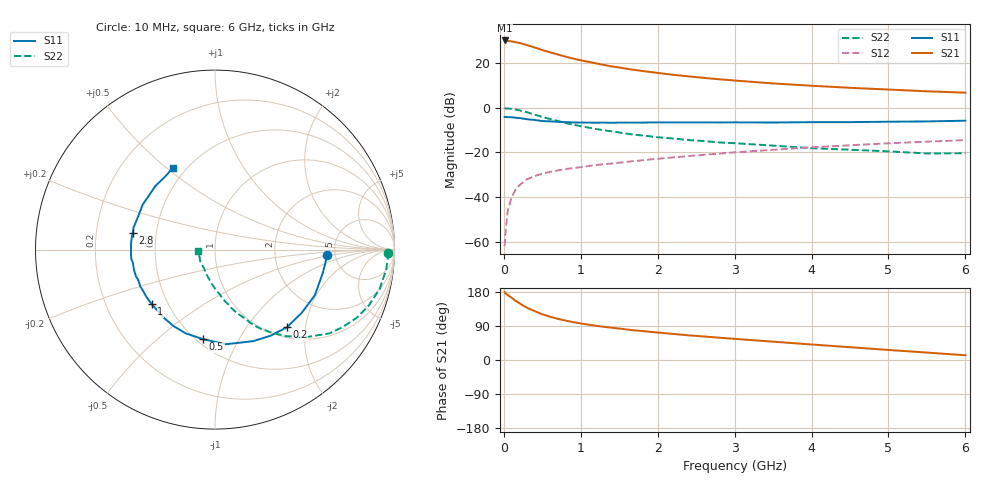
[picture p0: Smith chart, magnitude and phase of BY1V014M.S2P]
! SIEMENS Small Signal Semiconductors
! BFY420
! Si NPN RF SIEGET Grounded Emitter Transistor in MICRO-X
! VCE = 1 V  IC = 14 mA
! Common Emitter S-Parameters:  October  1996
# GHz  S  MA  R  50
!  f  S11  S21  S12  S22
! GHz  MAG  ANG  MAG  ANG  MAG  ANG  MAG  ANG
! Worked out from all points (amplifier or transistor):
!   36 points, 10 MHz to 6 GHz, reference 50 ohm
!   highest |S21| = 30.1 dB at 10 MHz (marker M1)
!   |S21| within 3 dB of that: start of sweep to 388.2 MHz
!   unconditionally stable (mu >= 1): 2.095 GHz to end of sweep
!   at 250 MHz: K = 0.25, MSG = 30.9 dB, |S12| = -33.3 dB
!   at 1.4 GHz: K = 0.86, MSG = 21.7 dB, |S12| = -25.0 dB
!   at 6 GHz: K = 1.10, MAG = 8.7 dB, |S12| = -14.5 dB
!   S11 on the Smith chart (normalised r, x): 10 MHz: 4.25, -0.41; 200 MHz: 1.19, -1.58; 500 MHz: 0.54, -0.72; 1 GHz: 0.41, -0.32; 2.8 GHz: 0.37, +0.09; 6 GHz: 0.43, +0.53
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0.01  0.6223 -2.7  31.9 179.1  0.0008 92.2  0.9613 -1.0
0.02  0.6218 -5.2  31.85 176.2  0.0015 90.9  0.9644 -2.4
0.05  0.6144 -12.3  31.03 171.6  0.0049 86.1  0.9605 -6.6
0.1  0.6118 -24.5  30.46 164.7  0.0098 79.0  0.9429 -13.5
0.15  0.598 -36.0  29.29 156.4  0.0144 73.1  0.9112 -20.1
0.2  0.5897 -47.2  28.18 150.4  0.0183 71.3  0.876 -25.8
0.25  0.5709 -57.3  26.64 143.7  0.0216 65.5  0.8303 -31.4
0.3  0.5527 -67.3  25.16 138.1  0.025 63.8  0.7904 -36.2
0.4  0.5308 -83.5  22.26 129.0  0.0296 58.3  0.7001 -44.3
0.5  0.5033 -97.5  19.46 120.6  0.0333 54.9  0.6229 -50.7
0.6  0.4943 -109.3  17.32 114.3  0.0368 53.0  0.5579 -55.9
0.7  0.4848 -118.4  15.51 108.7  0.0395 51.3  0.5043 -60.4
0.8  0.4749 -126.7  13.88 104.1  0.0423 49.9  0.4565 -64.0
1  0.4653 -139.3  11.48 96.5  0.0467 49.2  0.3862 -69.5
1.1  0.4642 -145.3  10.62 93.2  0.0496 49.6  0.359 -72.4
1.6  0.4653 -165.1  7.415 80.4  0.0616 49.3  0.263 -82.6
2.2  0.4683 180.0  5.443 68.8  0.0773 48.0  0.2048 -92.5
2.8  0.4675 168.3  4.327 58.9  0.0939 45.7  0.1671 -101.4
3.5  0.4664 156.0  3.492 48.4  0.1146 41.9  0.1417 -111.0
4.5  0.4754 140.7  2.784 33.8  0.1445 34.1  0.1149 -126.1
5.5  0.4928 124.2  2.327 19.6  0.1743 24.9  0.0947 -156.5
6  0.5122 117.3  2.17 12.5  0.1877 20.1  0.0959 -175.4
